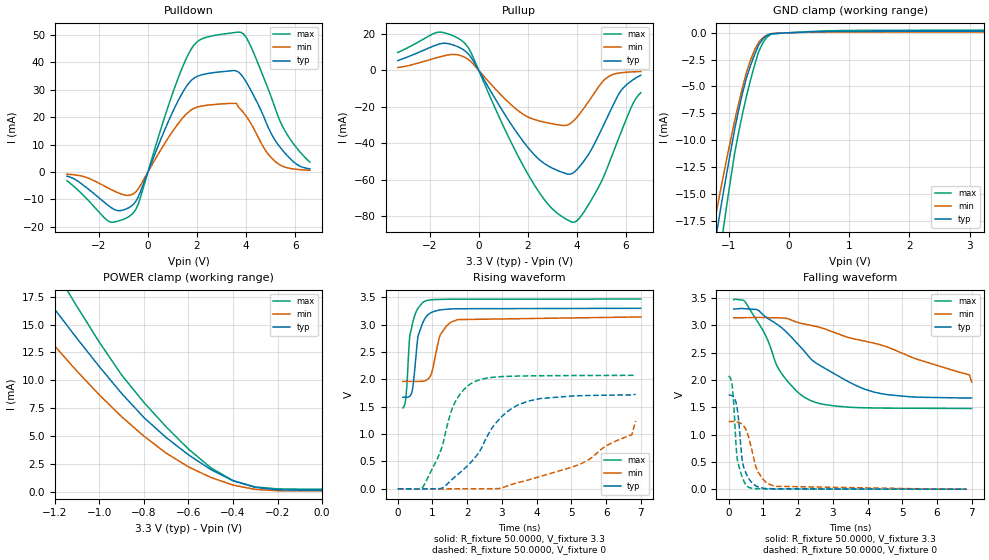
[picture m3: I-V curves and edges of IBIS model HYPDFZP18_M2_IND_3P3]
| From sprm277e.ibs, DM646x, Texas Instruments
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|   Model Cell HYPDFZP18_M2_IND_3P3
[Model]   HYPDFZP18_M2_IND_3P3
Model_type   I/O
Polarity   Non-Inverting
Enable   Active-Low
Vinl =  0.8V
Vinh =  2V
Cref =  10.0000pF
Rref =  50.0000
Vref =  1.5V
Vmeas =  1.65
C_comp   1.737544p   1.689782p   1.779236p
[Model Spec]
Vinl   0.8V   0.8V   0.8V
Vinh   2V   2V   2V
[Temperature Range]   25   125   -40
[Voltage Range]   3.3   3.14   3.47
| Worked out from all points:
|   slope of the pulldown table from 0 to 0.495 V, typ, clamps not added: 44 ohm
|   slope of the pullup table from 0 to 0.495 V, typ, clamps not added: 42.8 ohm
|   GND clamp passes 1 mA (typ) near -0.48 V on its own axis
|   POWER clamp passes 1 mA (typ) near -0.40 V on its own axis
|   rising waveform, R_fixture 50.0000, V_fixture 3.3: 20-80 % time 225ps typ, 314ps min, 183ps max; typ from 1.67 V to 3.3 V
|   rising waveform, R_fixture 50.0000, V_fixture 0: 20-80 % time 1.22ns typ, 2.51ns min, 686ps max; typ from 0 V to 1.73 V
|   falling waveform, R_fixture 50.0000, V_fixture 3.3: 20-80 % time 1.87ns typ, 3.46ns min, 1.01ns max; typ from 3.3 V to 1.67 V
|   falling waveform, R_fixture 50.0000, V_fixture 0: 20-80 % time 201ps typ, 362ps min, 163ps max; typ from 1.73 V to 0 V
[POWER_clamp]
|   voltage   I(typ)   I(min)   I(max)
-3.3V     84.8mA     64.02mA    102.5mA
-1.4V     21.98mA    17.81mA    26.65mA
-1.367V   21.02mA    17.01mA    25.52mA
-1.233V   17.27mA    13.85mA    21.02mA
-1.133V   14.62mA    11.57mA    17.71mA
-900mV    8.824mA    6.737mA    10.48mA
-800mV    6.66mA     4.988mA    8.019mA
-600mV    3.317mA    2.232mA    3.832mA
-500mV    1.995mA    1.287mA    2.162mA
-400mV    988uA      597.2uA    995.5uA
-300mV    389.7uA    206.1uA    428.6uA
0V        136.6uA    74.19uA    232.5uA
[Pulldown]
|   voltage   I(typ)   I(min)   I(max)
-3.3V     -1.512mA   -788.5uA   -3.181mA
-1.6V     -12.28mA   -5.92mA    -17.95mA
-700mV    -12.58mA   -8.352mA   -15.75mA
-400mV    -9.19mA    -6.204mA   -11.82mA
900mV     19.74mA    13.39mA    25.89mA
1.7V      32.7mA     22.18mA    43.75mA
2.2V      35.39mA    24.02mA    48.45mA
3.7V      36.3mA     23.5mA     50.91mA
4.2V      29.62mA    17.57mA    45.56mA
5.2V      11.29mA    3.715mA    22.78mA
5.7V      5.73mA     1.467mA    13.24mA
6.6V      1.129mA    616.6uA    3.569mA
[Pullup]
|   voltage   I(typ)   I(min)   I(max)
-3.3V     5.396mA    1.593mA    9.846mA
-1.7V     14.1mA     7.028mA    20.86mA
-600mV    11.14mA    7.391mA    15.31mA
1.3V      -29.12mA   -18.58mA   -38.91mA
2.2V      -45.34mA   -26.59mA   -61.37mA
3V        -53.59mA   -29.28mA   -75.94mA
3.8V      -56.59mA   -28.4mA    -83.18mA
4.3V      -49.37mA   -20.37mA   -77.33mA
5.2V      -26.74mA   -4.177mA   -54.59mA
5.8V      -10.99mA   -1.259mA   -33.78mA
6.3V      -4.974mA   -743uA     -17.68mA
6.6V      -2.652mA   -591.1uA   -12.21mA
[GND_clamp]
|   voltage   I(typ)   I(min)   I(max)
-3.3V     -103.4mA   -79.14mA   -123mA
-1.3V     -22.44mA   -19.56mA   -26.87mA
-1.233V   -19.98mA   -17.6mA    -24.16mA
-1.167V   -17.61mA   -15.65mA   -21.47mA
-1.1V     -15.33mA   -13.72mA   -18.81mA
-1.033V   -13.19mA   -11.85mA   -16.2mA
-900mV    -9.067mA   -8.253mA   -11.26mA
-700mV    -4.153mA   -3.637mA   -5.861mA
-500mV    -1.132mA   -881.2uA   -1.769mA
-366.7mV  -266uA     -229.7uA   -429.4uA
633.3mV   111.8uA    63.12uA    175.1uA
3.233V    136.4uA    76.57uA    231.4uA
[Ramp]
| variable   typ   min   max
dV/dt_f 0.98668153/1.8967395n 0.74627188/3.6601637n  1.2041177/1.0125075n
dV/dt_r  1.0398649/1.2293447n 0.75385023/2.5950738n   1.249285/0.68605478n
R_load = 50
[Rising Waveform]
R_fixture = 50.0000
V_fixture = 3.3
V_fixture_min = 3.14
V_fixture_max = 3.47
|   time   V(typ)   V(min)   V(max)
147.1ps   1.672V     1.962V     1.476V
229.8ps   1.672V     1.962V     1.652V
359.3ps   1.701V     1.962V     2.836V
442.2ps   1.898V     1.962V     3.063V
581.7ps   2.773V     1.962V     3.297V
771.1ps   3.098V     1.97V      3.424V
970ps     3.221V     2.106V     3.453V
1.233ns   3.268V     2.822V     3.459V
1.723ns   3.289V     3.091V     3.463V
6.996ns   3.297V     3.138V     3.466V
[Rising Waveform]
R_fixture = 50.0000
V_fixture = 0
V_fixture_min = 0
V_fixture_max = 0
|   time   V(typ)   V(min)   V(max)
0s        44.39uV    22.93uV    73.1uV
732ps     -3.074mV   -224.5uV   40.56mV
1.238ns   5.121mV    -4.24mV    701.7mV
1.617ns   201mV      -843.5uV   1.538V
2.216ns   563.2mV    35.14uV    1.958V
2.811ns   1.19V      1.708mV    2.041V
3.462ns   1.531V     112.1mV    2.059V
5.356ns   1.701V     480.9mV    2.069V
6.739ns   1.714V     986.7mV    2.071V
6.849ns   1.725V     1.238V     2.072V
[Falling Waveform]
R_fixture = 50.0000
V_fixture = 3.3
V_fixture_min = 3.14
V_fixture_max = 3.47
|   time   V(typ)   V(min)   V(max)
147.1ps   3.297V     3.138V     3.466V
452.9ps   3.305V     3.14V      3.446V
853.5ps   3.275V     3.145V     3.048V
1.096ns   3.14V      3.141V     2.772V
1.478ns   2.98V      3.136V     2.164V
1.92ns    2.706V     3.068V     1.819V
2.324ns   2.417V     3.005V     1.634V
4.198ns   1.776V     2.671V     1.486V
6.939ns   1.669V     2.091V     1.478V
6.996ns   1.672V     1.962V     1.476V
[Falling Waveform]
R_fixture = 50.0000
V_fixture = 0
V_fixture_min = 0
V_fixture_max = 0
|   time   V(typ)   V(min)   V(max)
0s        1.725V     1.238V     2.072V
74.02ps   1.718V     1.239V     1.999V
112.8ps   1.705V     1.239V     1.846V
220.4ps   1.564V     1.234V     757.4mV
256ps     1.435V     1.229V     526.6mV
401.9ps   492mV      1.182V     206.9mV
581ps     190.6mV    941.5mV    33.36mV
834.5ps   44.09mV    330.3mV    7.838mV
1.327ns   6.927mV    52.3mV     2.696mV
6.849ns   44.39uV    22.93uV    73.1uV
